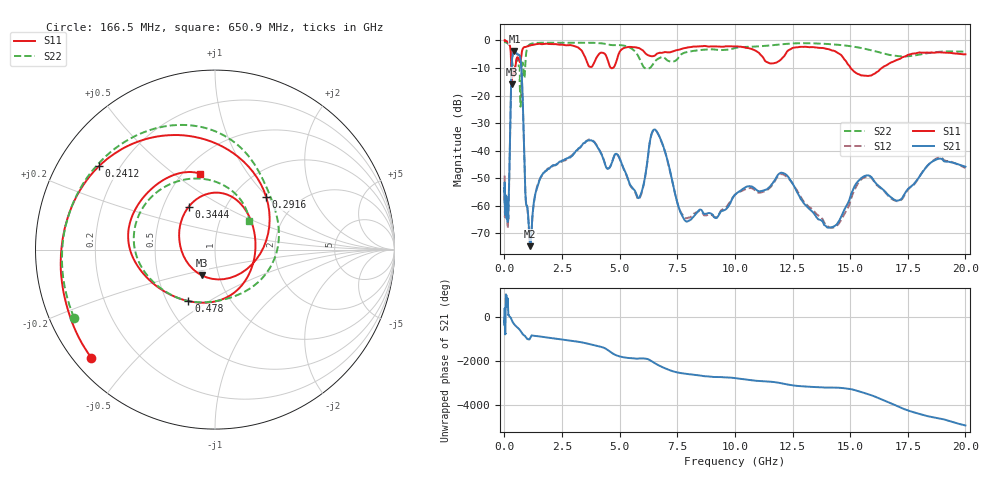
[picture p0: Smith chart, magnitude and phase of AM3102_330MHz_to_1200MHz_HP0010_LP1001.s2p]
! Date/Time: Tue, Sep 11, 2018 5:11 PM
! Network Analyzer: Agilent Technologies E8362B Rev: A.07.50.63
! Sweep from 0.010 to 20.000 GHz, 1601 Points, Sweep Type: LOG
! Power Supply: 4.950 V, 0.001 A
# Hz S DB R 50
!freq MagS11 AngS11 MagS21 AngS21 MagS12 AngS12 MagS22 AngS22
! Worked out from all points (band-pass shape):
!   1601 points, 10 MHz to 20 GHz, reference 50 ohm
!   highest |S21| = -3.80 dB at 438.8 MHz (marker M1); lowest = -74.6 dB at 1.113 GHz (marker M2)
!   |S21| within 3 dB of the highest: 333 MHz to 702.9 MHz (369.9 MHz wide, 71.4 % of centre)
!   lowest |S11| = -15.8 dB at 319.2 MHz (marker M3), VSWR 1.38, Z = 41.5 - j12.2 ohm
!   |S11| at or under -10 dB: 298.1 MHz to 357.8 MHz (59.7 MHz wide, 18.2 % of centre); 364.8 MHz to 474.9 MHz (110.1 MHz wide, 26.2 % of centre); 15.03 GHz to 16.37 GHz (1.347 GHz wide, 8.58 % of centre)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
!   |S22| runs from -24.0 to -0.3 dB; largest |S21 - S12| = 0.012
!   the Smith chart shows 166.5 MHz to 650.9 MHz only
!   S11 on the Smith chart (normalised r, x): 166.5 MHz: 0.05, -0.38; 241.2 MHz: 0.12, +0.32; 291.6 MHz: 1.40, +0.98; 344.4 MHz: 0.67, +0.35; 478 MHz: 0.64, -0.41; 650.9 MHz: 0.60, +0.63
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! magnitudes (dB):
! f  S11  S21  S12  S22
! 10 MHz  0.0  -52.4  -49.0  -0.3
! 35.55 MHz  0.0  -62.6  -59.3  -0.5
! 126.4 MHz  -0.4  -62.3  -62.5  -1.0
! 166.5 MHz  -0.8  -64.1  -65.7  -1.2
! 241.2 MHz  -2.0  -36.8  -37.1  -1.8
! 291.6 MHz  -7.8  -15.4  -15.5  -3.5
! 319.2 MHz  -15.8  -8.4  -8.4  -6.2
! 344.4 MHz  -11.0  -6.0  -6.1  -8.1
! 438.8 MHz  -11.9  -3.8  -3.9  -10.2
! 447.2 MHz  -11.5  -3.8  -3.9  -9.8
! 478 MHz  -9.8  -3.9  -4.0  -8.6
! 650.9 MHz  -7.3  -5.3  -5.4  -12.1
! 702.3 MHz  -7.5  -6.8  -6.8  -24.0
! 1.113 GHz  -1.8  -74.6  -73.9  -1.4
! 1.59 GHz  -1.3  -49.3  -49.5  -0.8
! 3.739 GHz  -9.6  -36.2  -35.9  -0.8
! 5.652 GHz  -2.4  -54.4  -54.8  -3.8
! 6.549 GHz  -5.3  -32.4  -32.5  -7.4
! 7.958 GHz  -2.5  -65.6  -64.4  -4.1
! 12.03 GHz  -6.6  -48.0  -48.5  -1.4
! 14.21 GHz  -3.6  -67.7  -68.0  -1.4
! 20 GHz  -5.0  -45.8  -46.2  -4.0
